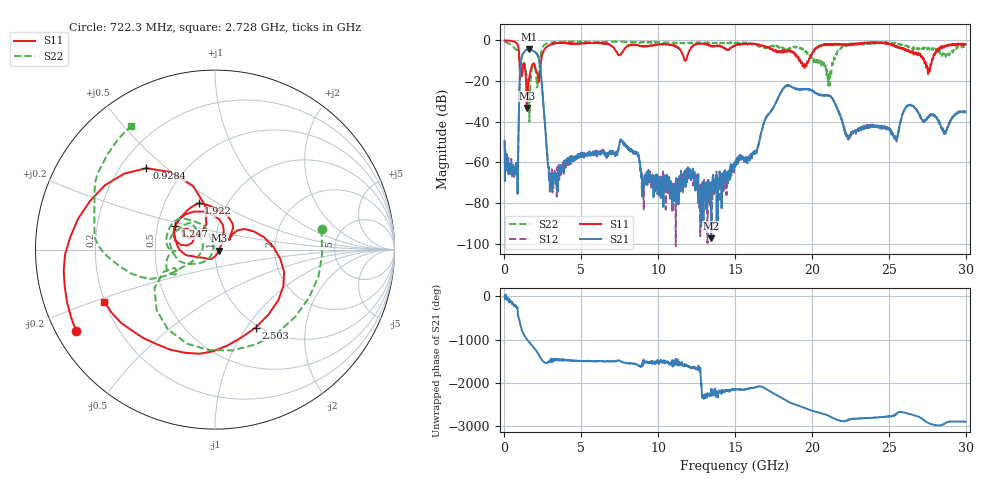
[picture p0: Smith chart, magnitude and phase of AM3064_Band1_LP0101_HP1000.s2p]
# Hz S DB R 50.0
!freq dBS11 angS11 dBS21 angS21 dBS12 angS12 dBS22 angS22
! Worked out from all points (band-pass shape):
!   1600 points, 10 MHz to 29.98 GHz, reference 50 ohm
!   highest |S21| = -4.37 dB at 1.584 GHz (marker M1); lowest = -97.4 dB at 13.45 GHz (marker M2)
!   |S21| within 3 dB of the highest: 1.153 GHz to 2.163 GHz (1.01 GHz wide, 60.9 % of centre)
!   lowest |S11| = -33.2 dB at 1.453 GHz (marker M3), VSWR 1.04, Z = 52.1 - j0.67 ohm
!   |S11| at or under -10 dB: 973.7 MHz to 2.387 GHz (1.413 GHz wide, 84.1 % of centre); 19.25 GHz to 19.79 GHz (542.9 MHz wide, 2.78 % of centre); 27.3 GHz to 27.79 GHz (494.9 MHz wide, 1.8 % of centre)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
!   |S22| runs from -40.0 to -0.4 dB; largest |S21 - S12| = 0.0083
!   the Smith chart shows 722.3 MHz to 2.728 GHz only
!   S11 on the Smith chart (normalised r, x): 722.3 MHz: 0.06, -0.27; 928.4 MHz: 0.31, +0.43; 1.247 GHz: 0.62, +0.17; 1.922 GHz: 0.74, +0.41; 2.503 GHz: 0.96, -1.10; 2.728 GHz: 0.20, -0.22
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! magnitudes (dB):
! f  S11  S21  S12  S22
! 10 MHz  0.0  -49.4  -49.4  -0.4
! 722.3 MHz  -0.9  -62.4  -65.0  -4.4
! 928.4 MHz  -4.5  -39.2  -39.2  -6.6
! 1.247 GHz  -11.7  -6.1  -6.0  -11.1
! 1.453 GHz  -33.2  -4.6  -4.5  -17.1
! 1.584 GHz  -19.6  -4.4  -4.4  -27.0
! 1.922 GHz  -11.3  -5.5  -5.4  -12.2
! 2.503 GHz  -6.2  -28.2  -28.1  -3.1
! 2.728 GHz  -3.3  -50.4  -50.8  -1.6
! 3.046 GHz  -1.9  -72.9  -68.7  -1.1
! 5.015 GHz  -1.4  -56.9  -56.7  -0.7
! 7.676 GHz  -5.8  -49.7  -49.7  -0.7
! 10 GHz  -2.1  -67.6  -67.5  -1.0
! 13.45 GHz  -2.6  -97.4  -69.0  -1.1
! 15 GHz  -2.5  -61.9  -59.4  -1.4
! 18.23 GHz  -5.6  -22.8  -22.7  -4.4
! 19.99 GHz  -7.2  -24.6  -24.6  -9.1
! 21.12 GHz  -1.7  -27.4  -27.2  -17.3
! 22.35 GHz  -1.9  -47.8  -47.2  -2.1
! 25 GHz  -1.4  -43.7  -43.4  -1.2
! 27.56 GHz  -16.5  -37.6  -38.0  -3.7
! 29.98 GHz  -1.8  -35.0  -35.3  -2.9
